PROGRAM move_prg
VAR
	meshod_table : ARRAY [0..8] OF STRING := [
		'Origin Switch',
		'Origin Switch + Z Phase',
		'Limit Switch',
		'LIMIT Switch + Z Phase',
		'Z Phase',
		'Torque LIMIT',
		'Torque LIMIT + Z Phase',
		'Set Origin'];
	dir_table : ARRAY [0..1] OF STRING := ['Negative Direction','Positive Direction'];

	target_pos: DINT;
	target_pos_g: DINT :=100000;
	target_pos_push: DINT :=100000;
	pos_back: DINT;

	stop_mode: BOOL;
	non_stop_mode: BOOL;
	
	abs_move: BOOL;
	dec_move: BOOL;
	inc_move: BOOL;
	minus_jog: BOOL;
	plus_jog: BOOL;
	
	move_r: BOOL;
	TON_0: TON;
	
	move_mode: UINT;
	start: UINT;
	standby: BOOL;
	TON_1: TON;
	stop_mode_r: BOOL;
	non_stop_mode_r: BOOL;
	
	org_method: BYTE :=0;
	org_dir: BYTE :=0;
	homing_method: SINT;
	home_sw: BOOL;
	
	SDO_Write01: FB_EcCoESdoWrite;
	
	TON_2: TON;
	write_set: BOOL;
	writeindex: WORD;
	writesubindex: BYTE;
	writevalu: UDINT;
	dint_writevalu: DINT;
	
	search_speed: UDINT :=1000;						//Object 6099h 2h: Homing Speeds(SUbIndex:1h Search Speed)
	homing_speed: UDINT :=5000;						//Object 6099h 1h: Homing Speeds(SUbIndex:2h Speed)
	homing_acceleration: UDINT :=100000;			//Object 609Ah: Homing Acceleration
	home_sel: WORD := 0;
	CTU_0: CTU;
END_VAR
VAR // added by the converter: edge detectors and wires of the graphical bodies
    _w1, _w2, _w3, _w4, _w5, _w6, _w7, _w8, _w9, _w10, _w11, _w12, _w13 : BOOL;
END_VAR

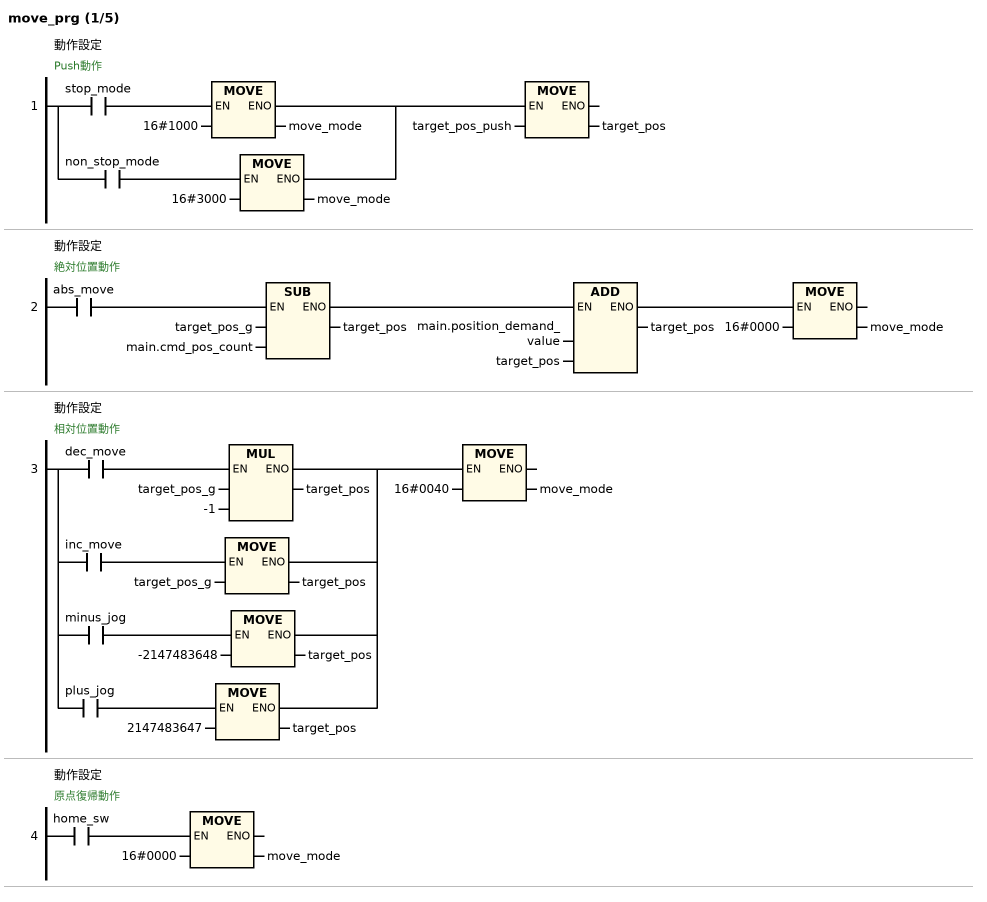
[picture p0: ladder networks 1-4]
// NETWORK 1: 動作設定
// Push動作
_w1 := stop_mode;
IF _w1 THEN move_mode := 16#1000; END_IF
_w2 := non_stop_mode;
IF _w2 THEN move_mode := 16#3000; END_IF
IF _w1 OR _w2 THEN target_pos := target_pos_push; END_IF

// NETWORK 2: 動作設定
// 絶対位置動作
_w3 := abs_move;
IF _w3 THEN target_pos := target_pos_g - main.cmd_pos_count; END_IF
IF _w3 THEN target_pos := main.position_demand_value + target_pos; END_IF
IF _w3 THEN move_mode := 16#0000; END_IF

// NETWORK 3: 動作設定
// 相対位置動作
_w4 := dec_move;
IF _w4 THEN target_pos := target_pos_g * -1; END_IF
_w5 := inc_move;
IF _w5 THEN target_pos := target_pos_g; END_IF
_w6 := minus_jog;
IF _w6 THEN target_pos := -2147483648; END_IF
_w7 := plus_jog;
IF _w7 THEN target_pos := 2147483647; END_IF
IF _w4 OR _w5 OR _w6 OR _w7 THEN move_mode := 16#0040; END_IF

// NETWORK 4: 動作設定
// 原点復帰動作
IF home_sw THEN move_mode := 16#0000; END_IF

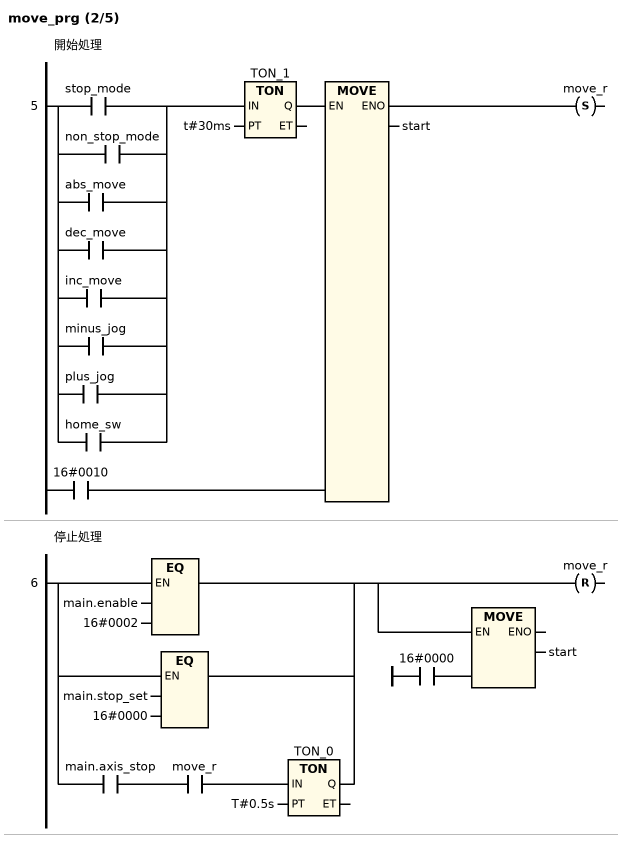
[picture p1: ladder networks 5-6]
// NETWORK 5: 開始処理
TON_1(IN := stop_mode OR non_stop_mode OR abs_move OR dec_move OR inc_move OR minus_jog OR plus_jog OR home_sw, PT := t#30ms); // TON
_w8 := TON_1.Q;
IF _w8 THEN start := 16#0010; END_IF
move_r S= _w8;

// NETWORK 6: 停止処理
TON_0(IN := main.axis_stop AND move_r, PT := T#0.5s); // TON
_w9 := main.enable = 16#0002 OR main.stop_set = 16#0000 OR TON_0.Q;
move_r R= _w9;
IF _w9 THEN start := 16#0000; END_IF

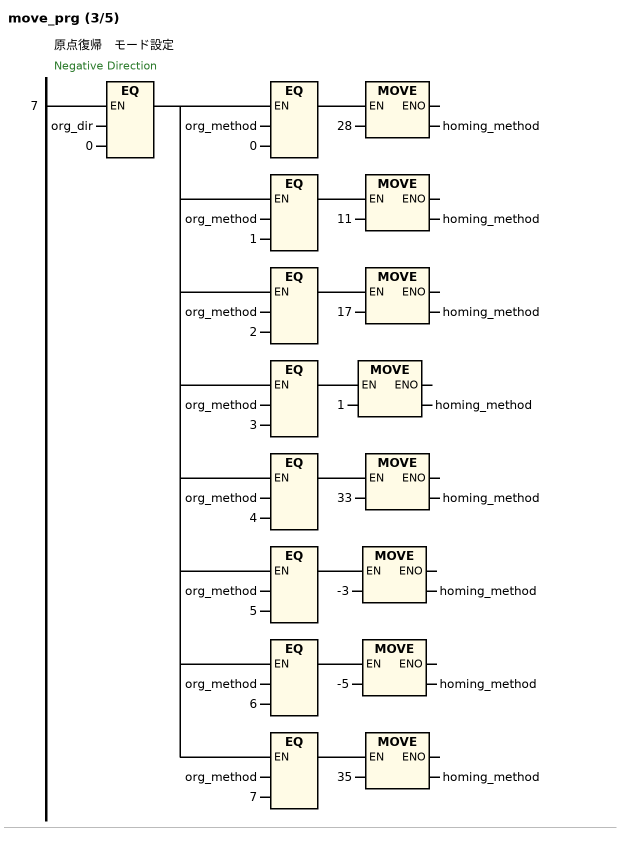
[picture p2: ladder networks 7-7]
// NETWORK 7: 原点復帰 モード設定
// Negative Direction
_w10 := org_dir = 0;
IF _w10 AND org_method = 0 THEN homing_method := 28; END_IF
IF _w10 AND org_method = 1 THEN homing_method := 11; END_IF
IF _w10 AND org_method = 2 THEN homing_method := 17; END_IF
IF _w10 AND org_method = 3 THEN homing_method := 1; END_IF
IF _w10 AND org_method = 4 THEN homing_method := 33; END_IF
IF _w10 AND org_method = 5 THEN homing_method := -3; END_IF
IF _w10 AND org_method = 6 THEN homing_method := -5; END_IF
IF _w10 AND org_method = 7 THEN homing_method := 35; END_IF

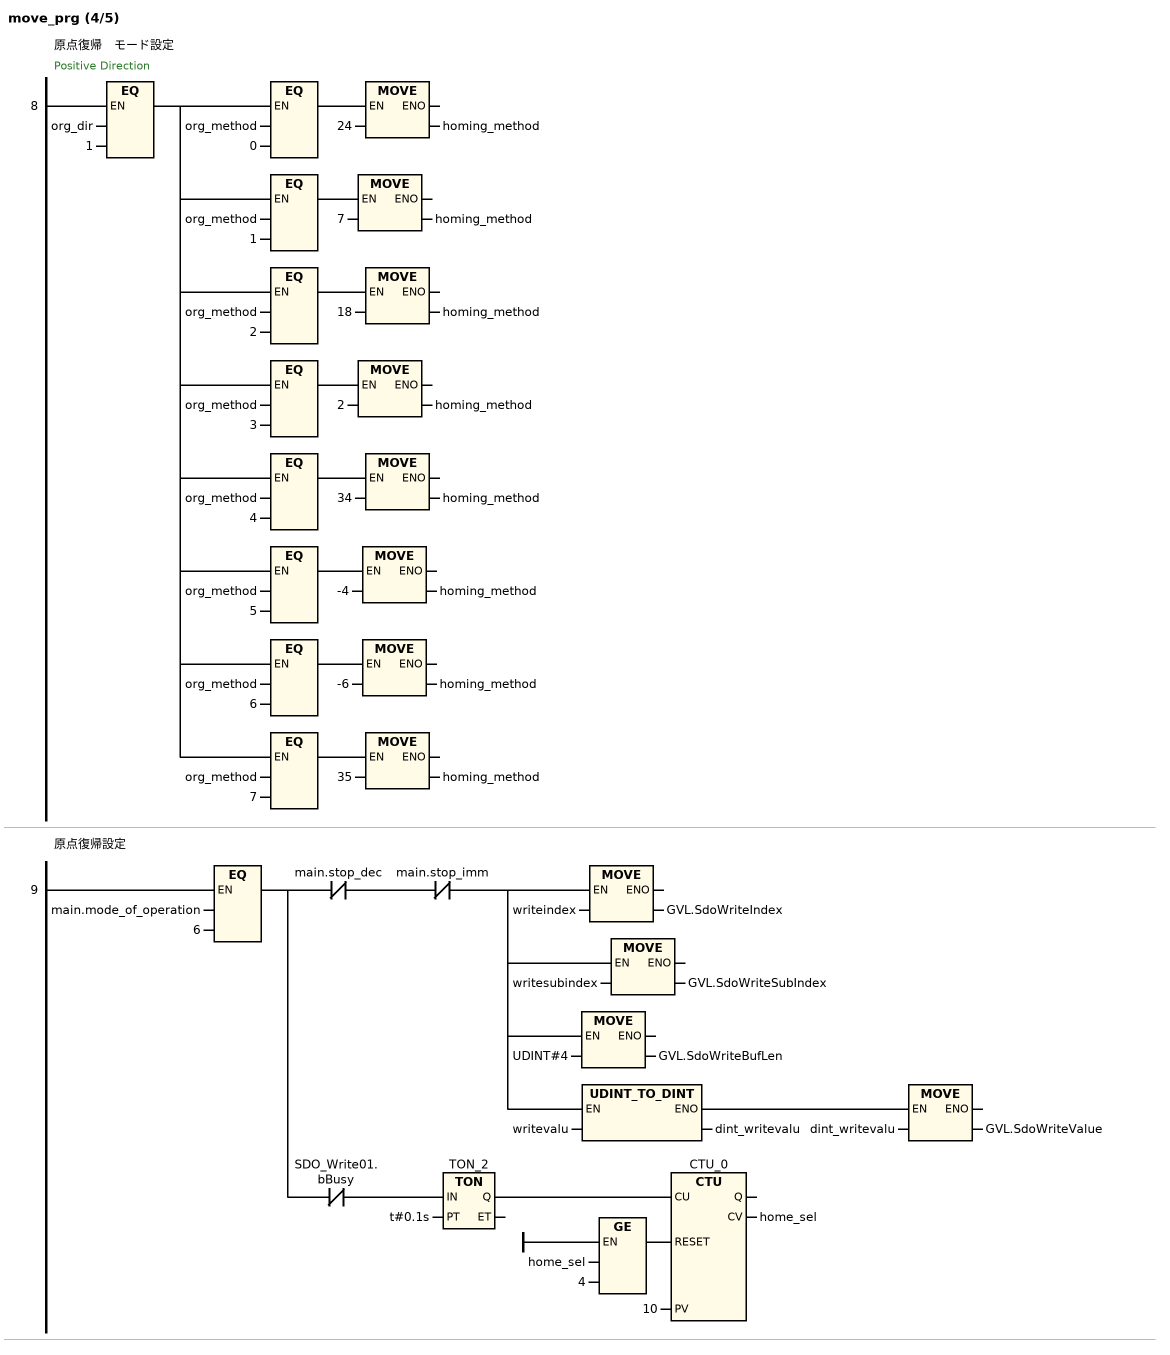
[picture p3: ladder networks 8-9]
// NETWORK 8: 原点復帰 モード設定
// Positive Direction
_w11 := org_dir = 1;
IF _w11 AND org_method = 0 THEN homing_method := 24; END_IF
IF _w11 AND org_method = 1 THEN homing_method := 7; END_IF
IF _w11 AND org_method = 2 THEN homing_method := 18; END_IF
IF _w11 AND org_method = 3 THEN homing_method := 2; END_IF
IF _w11 AND org_method = 4 THEN homing_method := 34; END_IF
IF _w11 AND org_method = 5 THEN homing_method := -4; END_IF
IF _w11 AND org_method = 6 THEN homing_method := -6; END_IF
IF _w11 AND org_method = 7 THEN homing_method := 35; END_IF

// NETWORK 9: 原点復帰設定
_w12 := main.mode_of_operation = 6;
_w13 := _w12 AND NOT main.stop_dec AND NOT main.stop_imm;
IF _w13 THEN GVL.SdoWriteIndex := writeindex; END_IF
IF _w13 THEN GVL.SdoWriteSubIndex := writesubindex; END_IF
IF _w13 THEN GVL.SdoWriteBufLen := UDINT#4; END_IF
IF _w13 THEN dint_writevalu := UDINT_TO_DINT(writevalu); END_IF
IF _w13 THEN GVL.SdoWriteValue := dint_writevalu; END_IF
TON_2(IN := _w12 AND NOT SDO_Write01.bBusy, PT := t#0.1s); // TON
CTU_0(CU := TON_2.Q, RESET := home_sel >= 4, PV := 10, CV => home_sel); // CTU

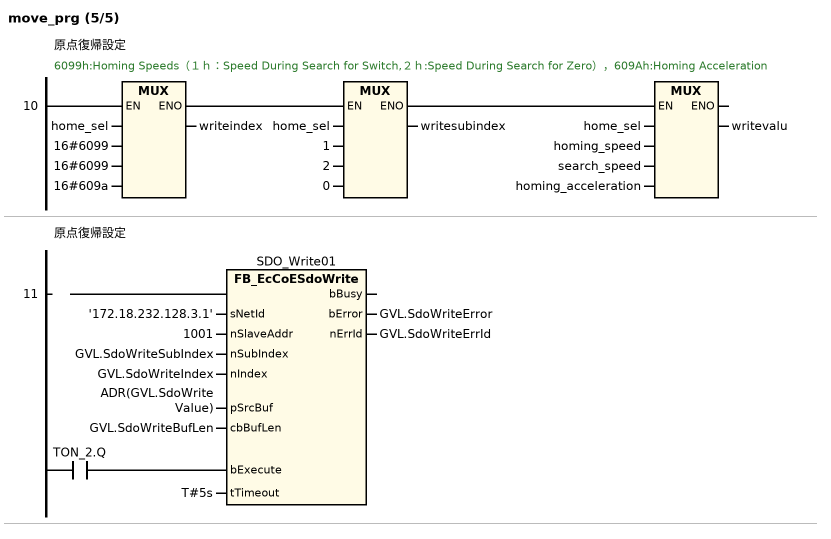
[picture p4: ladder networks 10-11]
// NETWORK 10: 原点復帰設定
// 6099h:Homing Speeds（１ｈ：Speed During Search for Switch,２ｈ:Speed During Search for Zero），609Ah:Homing Acceleration
writeindex := MUX(home_sel, 16#6099, 16#6099, 16#609a);
writesubindex := MUX(home_sel, 1, 2, 0);
writevalu := MUX(home_sel, homing_speed, search_speed, homing_acceleration);

// NETWORK 11: 原点復帰設定
SDO_Write01(
    sNetId := '172.18.232.128.3.1',
    nSlaveAddr := 1001,
    nSubIndex := GVL.SdoWriteSubIndex,
    nIndex := GVL.SdoWriteIndex,
    pSrcBuf := ADR(GVL.SdoWriteValue),
    cbBufLen := GVL.SdoWriteBufLen,
    bExecute := TON_2.Q,
    tTimeout := T#5s,
    bError => GVL.SdoWriteError,
    nErrId => GVL.SdoWriteErrId); // FB_EcCoESdoWrite

END_PROGRAM
